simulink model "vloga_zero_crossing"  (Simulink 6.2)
settings: Solver=ode45  StartTime=0.0  StopTime=2  RelTol=1e-5

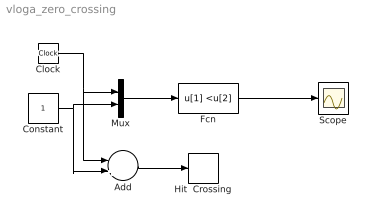
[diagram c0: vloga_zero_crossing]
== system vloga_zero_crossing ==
  Add : Sum  Inputs=-+  OutScaling=2^-10
  Clock : Clock
  Constant : Constant
  Fcn : Fcn  Expr=u[1] <u[2]
  Hit  Crossing : HitCross
  Mux : Mux  Inputs=2
  Scope : Scope
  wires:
  Clock/1 -> Mux/1, Add/1
  Constant/1 -> Mux/2, Add/2
  Mux/1 -> Fcn/1
  Fcn/1 -> Scope/1
  Add/1 -> Hit  Crossing/1
